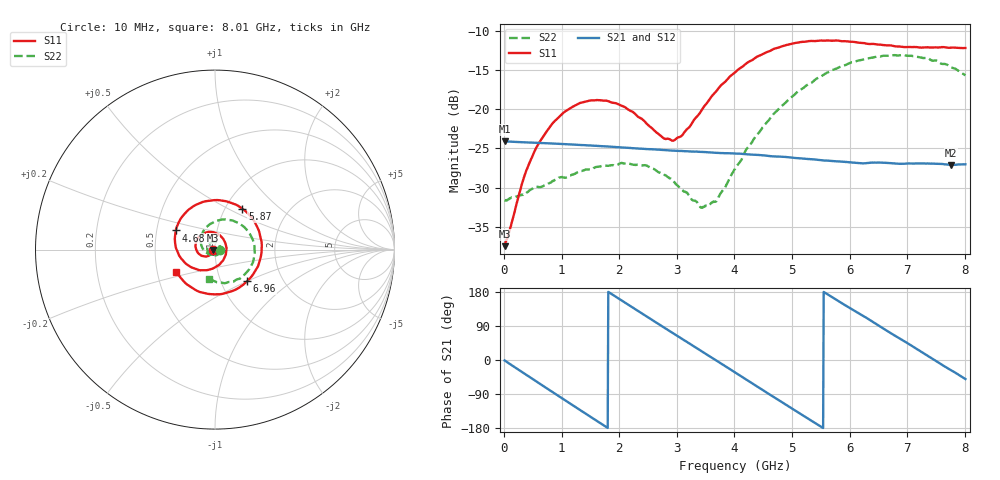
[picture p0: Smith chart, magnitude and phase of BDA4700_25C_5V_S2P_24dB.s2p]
!Agilent Technologies,E5071B,MY42404982,A.09.10
!Date: Mon Oct 20 13:38:31 2025
!Data & Calibration Information:
!Freq	S11:SOLT2(ON)	S21:SOLT2(ON)	S12:SOLT2(ON)	S22:SOLT2(ON)
# Hz S RI R 50
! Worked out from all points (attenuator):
!   801 points, 10 MHz to 8.01 GHz, reference 50 ohm
!   highest |S21| = -24.08 dB at 10 MHz (marker M1); lowest = -27.1 dB at 7.76 GHz (marker M2)
!   lowest |S11| = -37.5 dB at 10 MHz (marker M3), VSWR 1.03, Z = 48.7 - j0.149 ohm
!   |S11| at or under -10 dB: start of sweep to end of sweep
!   |S22| runs from -32.6 to -13.0 dB; largest |S21 - S12| = 0.00049
!   S11 on the Smith chart (normalised r, x): 10 MHz: 0.97, -0.00; 4.68 GHz: 0.63, +0.14; 5.87 GHz: 1.20, +0.59; 6.96 GHz: 1.33, -0.50; 8.01 GHz: 0.63, -0.16
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1e7  -0.0132 -0.00153  0.0625 -0.00133  0.0625 -0.0014  0.0262 -0.000835
3.5e8  -0.0251 -0.0273  0.0501 -0.0358  0.0501 -0.0358  0.0223 -0.0178
5.7e8  -0.0436 -0.038  0.0328 -0.0516  0.0328 -0.0516  0.0143 -0.0286
8.8e8  -0.0776 -0.0328  0.00168 -0.0604  0.00169 -0.0605  -0.00689 -0.0346
1.35e9  -0.1091 0.0197  -0.0418 -0.0419  -0.0418 -0.0419  -0.0362 -0.0178
1.97e9  -0.053 0.0948  -0.0552 0.0158  -0.0551 0.0158  -0.0341 0.028
2.45e9  0.0284 0.0781  -0.0257 0.0495  -0.0257 0.0496  -0.0028 0.0439
2.68e9  0.0555 0.0422  -0.00503 0.055  -0.00503 0.055  0.0132 0.0374
2.96e9  0.0618 -0.0151  0.0201 0.0505  0.0201 0.0505  0.0258 0.0224
3.44e9  -0.00173 -0.1004  0.0495 0.0202  0.0496 0.0201  0.0186 -0.0144
3.69e9  -0.0637 -0.115  0.0527 -0.0017  0.0528 -0.00182  0.000454 -0.0259
4.01e9  -0.1487 -0.0879  0.044 -0.0282  0.044 -0.0281  -0.0325 -0.0259
4.38e9  -0.2161 0.00488  0.0188 -0.0476  0.0188 -0.0477  -0.0682 0.00372
4.68e9  -0.2191 0.1067  -0.00639 -0.0496  -0.0063 -0.0497  -0.0801 0.0481
5.35e9  -0.0472 0.2701  -0.0455 -0.0153  -0.0455 -0.0153  -0.0157 0.1483
5.87e9  0.1522 0.227  -0.0399 0.0235  -0.0399 0.0235  0.1007 0.1608
6.26e9  0.246 0.0997  -0.0184 0.0413  -0.018 0.0414  0.1817 0.1036
6.68e9  0.2455 -0.0769  0.0125 0.0437  0.0125 0.0437  0.2204 -0.000407
6.96e9  0.1786 -0.176  0.0298 0.0337  0.0299 0.0335  0.209 -0.0761
7.35e9  0.0275 -0.2486  0.0441 0.0091  0.0442 0.00904  0.1404 -0.1604
7.76e9  -0.1451 -0.2018  0.0393 -0.02  0.0394 -0.0201  0.0306 -0.1835
8.01e9  -0.215 -0.1226  0.0285 -0.0342  0.0286 -0.0342  -0.0312 -0.1621
